//{{V2}}
FUNCTION_BLOCK FB74
TITLE=Move to Target Position
//*****************************************************************************
//* maxon motor ag
//* R&D
//* all rights reserved
//*****************************************************************************
//* Summary:  Move point to point
//*
//* Remarks:
//*
//* Created under: STEP7 REV5.2+SP1
//*****************************************************************************
//* History:
//* 19.05.2004 | INA   first release
//*
//*
//*****************************************************************************
//


AUTHOR:INA
FAMILY:ProPosMo
NAME:MoveToPo
VERSION:00.01


VAR_INPUT
       Write:BOOL //A rising edge start the command
       NodeID:BYTE //Adress of the maxon device
       TargetPosition:DINT //Target Position
       Absolute:BOOL //TRUE starts an absolute, FALSE a relative movement
       Immediately:BOOL //TRUE starts immediately, FALSE waits to end of last positioning
END_VAR

VAR_OUTPUT
       Done:BOOL //Data valid flag is TRUE if data were available
       Err:BOOL //Error flag is TRUE if an Error has occured, see ErrNo for more details
       ErrNo:DINT //Contains detailed error information
END_VAR

VAR_IN_OUT
END_VAR

VAR
       xEdgeMerker:BOOL //Edge Merker
       xEdgeFlag:BOOL //Edge Flag
       xStep:INT
       xAbsolutePosition:WORD:=W#16#001F
       xRelativePosition:WORD:=W#16#005F
       xImmediatelyAbs:WORD:=W#16#003F
       xImmediatelyRel:WORD:=W#16#007F
END_VAR

VAR_TEMP
END_VAR
BEGIN

NETWORK
TITLE= Activate the service function
//{{a}}
//

// SDO Write "Move to Target Position"

       U    #Write
       FP   #xEdgeFlag                   // recognize a positiv edge of the Read signal
       =    #xEdgeMerker                 // and set the xEdgeMerker for one cycle to true

       L    #xStep
       L    0
       ==I
       U    #xEdgeMerker
       SPB  nstp                         // iStep = 1 -> fnc1

       L    #xStep                       // jump list
       SPL  List
       SPA  rdef
       SPA  fnc1
       SPA  fncE
List  :SPA  rdef

rdef  :NOP  0
       R    #Done                        // reset Done
       R    #Err                         // reset Error
       L    0
       T    #xStep                       // iStep = 0
       SPA  end

fnc1  :NOP  0
       CALL FC13
         NodeID:=#NodeID
         Index:=DW#16#0000607A
         SubIndex:=DW#16#00000000
         ValueIn:=#TargetPosition
         RET_VAL:=#Done
         Err:=#Err
         ErrNo:=#ErrNo

       L    1
       U    #Err
       SPB  fncE

       NOP  0
       L    1
       U    #Absolute
       SPBN rel

       L    1
       U    #Immediately
       SPBN immR

       CALL FC15                         // Abs + Immediately
         NodeID:=#NodeID
         Index:=DW#16#00006040
         SubIndex:=DW#16#00000000
         ValueIn:=#xImmediatelyAbs
         RET_VAL:=#Done
         Err:=#Err
         ErrNo:=#ErrNo

       L    1
       U    #Err
       SPB  fncE

       SPA  nstp                         // iStep = 2 -> fncE

       NOP  0
       CALL FC15                         // Abs + not Immediately
         NodeID:=#NodeID
         Index:=DW#16#00006040
         SubIndex:=DW#16#00000000
         ValueIn:=#xAbsolutePosition
         RET_VAL:=#Done
         Err:=#Err
         ErrNo:=#ErrNo

       L    1
       U    #Err
       SPB  fncE

       SPA  nstp                         // iStep = 2 -> fncE

rel   :NOP  0

       L    1
       U    #Immediately
       SPBN immR

       CALL FC15                         // Rel + immediately
         NodeID:=#NodeID
         Index:=DW#16#00006040
         SubIndex:=DW#16#00000000
         ValueIn:=#xImmediatelyRel
         RET_VAL:=#Done
         Err:=#Err
         ErrNo:=#ErrNo

       L    1
       U    #Err
       SPB  fncE

       SPA  nstp                         // iStep = 2 -> fncE

immR  :NOP  0
       CALL FC15                         // Rel + not immediately
         NodeID:=#NodeID
         Index:=DW#16#00006040
         SubIndex:=DW#16#00000000
         ValueIn:=#xRelativePosition
         RET_VAL:=#Done
         Err:=#Err
         ErrNo:=#ErrNo

       L    1
       U    #Err
       SPB  fncE

       SPA  nstp                         // iStep = 2 -> fncE

fncE  :NOP  0
       L    0
       T    #xStep
       SPA  end

nstp  :NOP  0
       L    #xStep
       INC            1
       T    #xStep

end   :NOP  0
END_FUNCTION_BLOCK
